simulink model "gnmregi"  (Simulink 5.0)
settings: Solver=ode45  StartTime=0.0  StopTime=Tstop  MaxStep=step_max  RelTol=1e-3
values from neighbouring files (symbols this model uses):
  CE = 2*pi*CM    (= 240.017678734)    [gnm_i.m]
  CM = 38.2    [gnm_i.m]
  IA_soll = 10    [gnmregi_i.m]
  int_regi = 0    [gnmregi_i.m]
  J = 0.012    [gnm_i.m]
  MW = 10    [gnmbeobreg_i.m]    (also in gnmbeob_i.m; gnmregn_i.m = 100; gnm_i.m = 0; lsg_gnmregnss_ini.m = 100)
  PsiN = 0.04    [gnm_i.m]
  RA = 0.250    (= 0.25)    [gnm_i.m]
  T_IAsoll = 0.05    [gnmregi_i.m]
  T_MW = 0.4    [gnmbeobreg_i.m]    (also in gnmbeob_i.m; gnmregn_i.m = 0.1; gnm_i.m = 0; lsg_gnmregnss_ini.m = 0.1)
  T_Ri = TA    [gnmregi_i.m]
  T_t = 0.0001    [gnmbeobreg_i.m]    (also in gnmbeob_i.m; gnmregi_i.m)
  TA = LA / RA    (= 0.016)    [gnm_i.m]
  V_Ri = LA / (2*T_t)    [gnmregi_i.m]

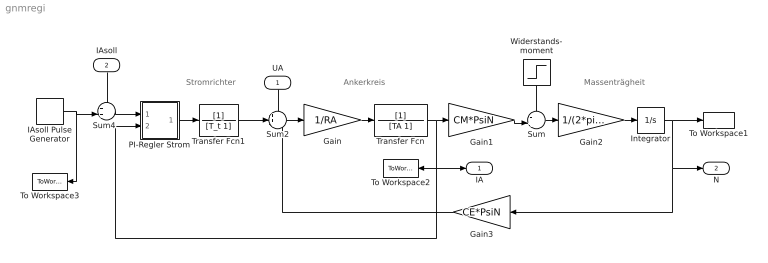
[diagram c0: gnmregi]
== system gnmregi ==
  note: Massenträgheit
  note: Ankerkreis
  note: Stromrichter
  UA : Inport  Orientation=down
  IAsoll : Inport  Orientation=down  Port=2  PortDimensions=1
  Gain : Gain  Gain=1/RA
  Gain1 : Gain  Gain=CM*PsiN
  Gain2 : Gain  Gain=1/(2*pi*J)
  Gain3 : Gain  Orientation=left  Gain=CE*PsiN
  IAsoll Pulse Generator : DiscretePulseGenerator  PulseType=Time based  Amplitude=IA_soll  Period=T_IAsoll  PulseWidth=50
  Integrator : Integrator
  PI-Regler Strom : Subsystem  mask(PI-Regler){V_R=V_Ri, T_n=T_Ri, int_R=int_regi}
      mask prompts: V_R "Verstärkungsfaktor V_R"; T_n "Nachstellzeit T_n"; int_R "Startwert Regler-Integrator"
      mask help: 1 + s*T_n 1 + s*T_n Übertragungsfunktion: G_R = V_R * ------------------ = K_R * ------------------ s*T_n s
  Sum : Sum  Inputs=-+|
  Sum2 : Sum  Inputs=++-
  Sum4 : Sum  Inputs=++|
  To Workspace1 : ToWorkspace  VariableName=N  SampleTime=-1  SaveFormat=Array
  To Workspace2 : ToWorkspace  VariableName=IA  SampleTime=-1  SaveFormat=Array
  To Workspace3 : ToWorkspace  VariableName=IAsoll  SampleTime=-1  SaveFormat=Array
  Transfer Fcn : TransferFcn  Denominator=[TA 1]
  Transfer Fcn1 : TransferFcn  Denominator=[T_t 1]
  Widerstands- moment : Step  Orientation=down  Time=T_MW  After=MW  SampleTime=0
  IA : Outport
  N : Outport  Port=2
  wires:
  PI-Regler Strom/1(Reglerausgang) -> Transfer Fcn1/1
  IAsoll/1 -> Sum4/1
  Sum4/1 -> PI-Regler Strom/1(Sollwert)
  Gain/1 -> Transfer Fcn/1
  Sum2/1 -> Gain/1
  Gain1/1 -> Sum/2
  Widerstands- moment/1 -> Sum/1
  Sum/1 -> Gain2/1
  Gain2/1 -> Integrator/1
  Integrator/1 -> To Workspace1/1, N/1, Gain3/1
  UA/1 -> Sum2/1
  Gain3/1 -> Sum2/3
  Transfer Fcn/1 -> Gain1/1, To Workspace2/1, IA/1, PI-Regler Strom/2(Istwert)
  Transfer Fcn1/1 -> Sum2/2
  IAsoll Pulse Generator/1 -> Sum4/2, To Workspace3/1

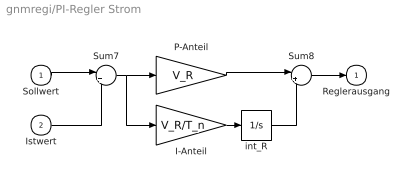
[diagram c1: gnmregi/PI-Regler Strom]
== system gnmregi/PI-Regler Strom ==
  Sollwert : Inport
  Istwert : Inport  Port=2
  I-Anteil : Gain  Gain=V_R/T_n
  P-Anteil : Gain  Gain=V_R
  Sum7 : Sum  Inputs=|+-
  Sum8 : Sum  Inputs=|++
  int_R : Integrator  InitialCondition=int_R
  Reglerausgang : Outport  InitialOutput=0
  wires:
  P-Anteil/1 -> Sum8/1
  I-Anteil/1 -> int_R/1
  int_R/1 -> Sum8/2
  Sum8/1 -> Reglerausgang/1
  Sum7/1 -> P-Anteil/1, I-Anteil/1
  Istwert/1 -> Sum7/2
  Sollwert/1 -> Sum7/1
